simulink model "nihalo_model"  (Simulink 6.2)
settings: Solver=ode45  StartTime=0.0  StopTime=10.0  RelTol=1e-3
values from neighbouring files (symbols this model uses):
  c = 1.96    [nihalom.m]
  g = 9.81    [nihalom.m]
  l = 9.81    [nihalom.m]
  m = 1    [nihalom.m]    (also in Razs_z_transm.m = sym('m','positive'); Primer_14_2.m = sym('m','positive'))
  x10 = pi    (= 3.14159265359)    [nihalom.m]
  x20 = -0.01    [nihalom.m]

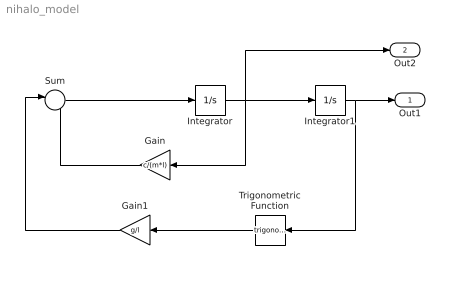
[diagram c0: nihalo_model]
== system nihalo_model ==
  Gain : Gain  Orientation=left  Gain=c/(m*l)
  Gain1 : Gain  Orientation=left  Gain=g/l
  Integrator : Integrator  InitialCondition=x20
  Integrator1 : Integrator  InitialCondition=x10
  Sum : Sum  Inputs=|--
  Trigonometric Function : Trigonometry  Orientation=left
  Out1 : Outport
  Out2 : Outport  Port=2
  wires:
  Sum/1 -> Integrator/1
  Integrator/1 -> Integrator1/1, Gain/1, Out2/1
  Integrator1/1 -> Trigonometric Function/1, Out1/1
  Trigonometric Function/1 -> Gain1/1
  Gain1/1 -> Sum/1
  Gain/1 -> Sum/2
